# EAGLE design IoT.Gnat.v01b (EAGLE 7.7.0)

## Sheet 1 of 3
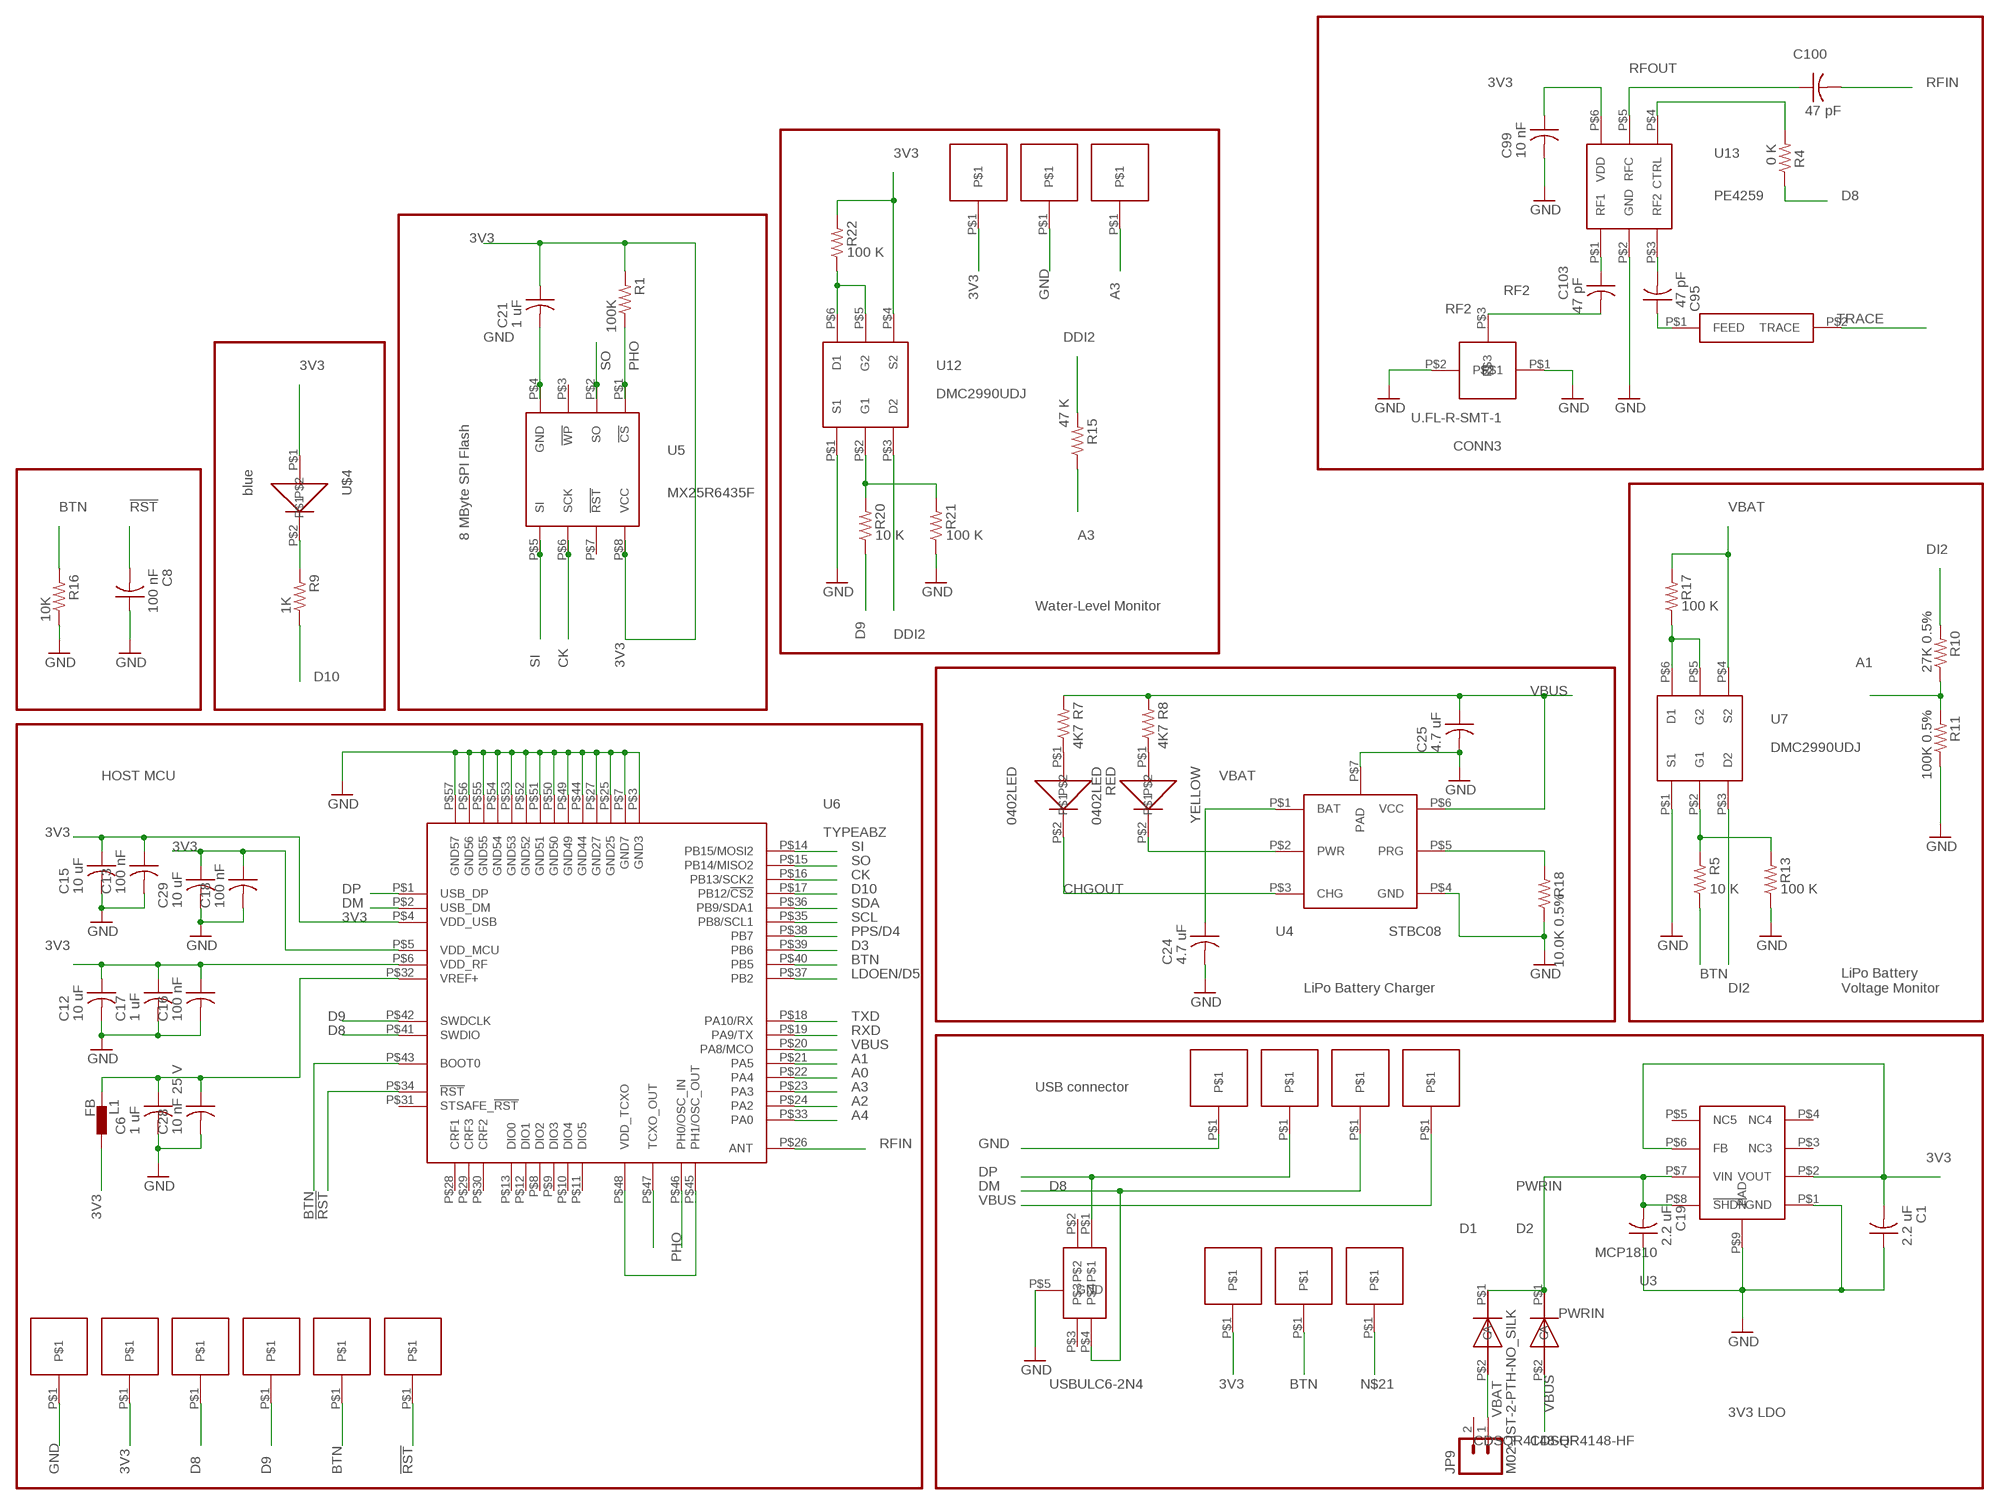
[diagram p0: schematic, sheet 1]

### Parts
C1  2.2 uF  C-US  [C0402_B]
C6  1 uF  C-US  [C0402_B]
C8  100 nF  C-US  [C0402_B]
C12  10 uF  C-US  [C0402_B]
C13  100 nF  C-US  [C0402_B]
C15  10 uF  C-US  [C0402_B]
C16  100 nF  C-US  [C0402_B]
C17  1 uF  C-US  [C0402_B]
C18  100 nF  C-US  [C0402_B]
C19  2.2 uF  C-US  [C0402_B]
C21  1 uF  C-US  [C0402_B]
C24  4.7 uF  C-US  [C0402_B]
C25  4.7 uF  C-US  [C0402_B]
C28  10 nF 25 V  C-US  [C0402_B]
C29  10 uF  C-US  [C0402_B]
C95  47 pF  C-US  [C0402_B]
C99  10 nF  C-US  [C0402_B]
C100  47 pF  C-US  [C0402_B]
C103  47 pF  C-US  [C0402_B]
CONN3  U.FL-R-SMT-1  [U.FL-R-SMT-1]
D1  CDSQR4148-HF  [CDSQR4148-HF]
D2  CDSQR4148-HF  [CDSQR4148-HF]
D8  USBULC6-2N4  [USBULC6-2N4]
JP9  M02-JST-2-PTH-NO_SILK  [JST-2-PTH-NS]
L1  FB  BLM15H  [0402]
R1  100K  R-US_  [R0402_B]
R4  0 K  R-US_  [R0402_B]
R5  10 K  R-US_  [R0402_B]
R7  4K7  R-US_  [R0402_B]
R8  4K7  R-US_  [R0402_B]
R9  1K  R-US_  [R0402_B]
R10  27K 0.5%  R-US_  [R0402_B]
R11  100K 0.5%  R-US_  [R0402_B]
R13  100 K  R-US_  [R0402_B]
R15  47 K  R-US_  [R0402_B]
R16  10K  R-US_  [R0402_B]
R17  100 K  R-US_  [R0402_B]
R18  10.0K 0.5%  R-US_  [R0402_B]
R20  10 K  R-US_  [R0402_B]
R21  100 K  R-US_  [R0402_B]
R22  100 K  R-US_  [R0402_B]
RED  0402LED  [0402LED]
U3  MCP1810  [MCP1810]
U4  STBC08  [STBC08]
U5  MX25R6435F  [MX25R6435F]
U6  TYPEABZ  [TYPEABZ]
U7  DMC2990UDJ  [DMC2990UDJ]
U12  DMC2990UDJ  [DMC2990UDJ]
U13  PE4259  [PE4259]
U$1  HN01  [HN01]
U$2  JOHANSON0900AT43A0070  [JOHANSON0900AT43A0070]
U$3  HN01  [HN01]
U$4  blue  0402LED  [0402LED]
U$6  HN01  [HN01]
U$7  HN01  [HN01]
U$8  HN01  [HN01]
U$9  HN01  [HN01]
U$10  HN01  [HN01]
U$11  HN01  [HN01]
U$12  HN01  [HN01]
U$13  HN01  [HN01]
U$14  HN01  [HN01]
U$15  HN01  [HN01]
U$16  HN01  [HN01]
U$17  HN01  [HN01]
U$18  HN01  [HN01]
U$19  HN01  [HN01]
YELLOW  0402LED  [0402LED]

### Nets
3V3: C1.2 C12.1 C13.1 C15.1 C16.1 C17.1 C18.1 C21.1 C29.1 C99.1 L1.2 R1.2 R22.2 U3.P$2(VOUT) U3.P$6(FB) U5.P$8(VCC) U6.P$4(VDD_USB) U6.P$5(VDD_MCU) U6.P$6(VDD_RF) U12.P$4(S2) U13.P$6(VDD) U$4.P$1 U$8.P$1 U$10.P$1 U$19.P$1 ; also sheet 2,3
!RST: C8.2 U6.P$34(!RST) U$9.P$1
A0: U6.P$22(PA4) ; also sheet 2
A1: R10.1 R11.2 U6.P$21(PA5)
A2: U6.P$24(PA2) ; also sheet 3
A3: R15.1 U6.P$23(PA3) U$12.P$1
A4: U6.P$33(PA0) ; also sheet 3
AREF: C6.1 C28.1 L1.1 U6.P$32(VREF+)
BTN: R5.1 R16.2 U6.P$40(PB5) U6.P$43(BOOT0) U$6.P$1 U$17.P$1
CHGOUT: RED.P$2 U4.P$3(CHG)
CK: U5.P$6(SCK) U6.P$16(PB13/SCK2)
D3: U6.P$39(PB6) ; also sheet 3
D8: R4.1 U6.P$41(SWDIO) U$1.P$1
D9: R20.1 U6.P$42(SWDCLK) U$3.P$1
D10: R9.1 U6.P$17(PB12/!CS2)
DDI2: R15.2 U12.P$3(D2)
DI2: R10.2 U7.P$3(D2)
DM: D8.P$4 U6.P$2(USB_DM) U$15.P$1
DP: D8.P$1 U6.P$1(USB_DP) U$14.P$1
GND: C1.1 C6.2 C8.1 C12.2 C13.2 C15.2 C16.2 C17.2 C18.2 C19.1 C21.2 C24.2 C25.2 C28.2 C29.2 C99.2 CONN3.P$1 CONN3.P$2 D8.P$5(GND) R11.1 R13.1 R16.1 R18.1 R21.1 U3.P$1(GND) U3.P$9(PAD) U4.P$4(GND) U4.P$7(PAD) U5.P$4(GND) U6.P$3(GND3) U6.P$7(GND7) U6.P$25(GND25) U6.P$27(GND27) U6.P$44(GND44) U6.P$49(GND49) U6.P$50(GND50) U6.P$51(GND51) U6.P$52(GND52) U6.P$53(GND53) U6.P$54(GND54) U6.P$55(GND55) U6.P$56(GND56) U6.P$57(GND57) U7.P$1(S1) U12.P$1(S1) U13.P$2(GND) U$7.P$1 U$11.P$1 U$13.P$1 ; also sheet 2,3
LDOEN/D5: U6.P$37(PB2) ; also sheet 2
N$2: U6.P$45(PH1/OSC_OUT) U6.P$48(VDD_TCXO)
N$3: R9.2 U$4.P$2
N$4: R20.2 R21.2 U12.P$2(G1)
N$7: U4.P$2(PWR) YELLOW.P$2
N$9: U6.P$47(TCXO_OUT)
N$10: R22.1 U12.P$5(G2) U12.P$6(D1)
N$12: R5.2 R13.2 U7.P$2(G1)
N$13: R17.1 U7.P$5(G2) U7.P$6(D1)
N$15: R7.1 RED.P$1
N$16: C95.1 U$2.P$1(FEED)
N$17: R8.1 YELLOW.P$1
N$18: C95.2 U13.P$3(RF2)
N$19: C103.1 U13.P$1(RF1)
N$21: U$18.P$1
N$22: R4.2 U13.P$4(CTRL)
N$27: R18.2 U4.P$5(PRG)
PHO: R1.1 U5.P$1(!CS) U6.P$46(PH0/OSC_IN)
PPS/D4: U6.P$38(PB7) ; also sheet 2
PWRIN: C19.2 D1.P$1(C) D2.P$1(C) U3.P$7(VIN) U3.P$8(!SHDN)
RF2: C103.2 CONN3.P$3
RFIN: C100.2 U6.P$26(ANT)
RFOUT: C100.1 U13.P$5(RFC)
RXD: U6.P$19(PA9/TX) ; also sheet 2
SCL: U6.P$35(PB8/SCL1) ; also sheet 3
SDA: U6.P$36(PB9/SDA1) ; also sheet 3
SI: U5.P$5(SI) U6.P$14(PB15/MOSI2)
SO: U5.P$2(SO) U6.P$15(PB14/MISO2)
TRACE: U$2.P$2(TRACE)
TXD: U6.P$18(PA10/RX) ; also sheet 2
VBAT: C24.1 D1.P$2(A) JP9.1 R17.2 U4.P$1(BAT) U7.P$4(S2)
VBUS: C25.1 D2.P$2(A) R7.2 R8.2 U4.P$6(VCC) U6.P$20(PA8/MCO) U$16.P$1
Unconnected: D8.P$2 D8.P$3 JP9.2 U3.P$3(NC3) U3.P$4(NC4) U3.P$5(NC5) U5.P$3(!WP) U5.P$7(!RST) U6.P$8(DIO2) U6.P$9(DIO3) U6.P$10(DIO4) U6.P$11(DIO5) U6.P$12(DIO1) U6.P$13(DIO0) U6.P$28(CRF1) U6.P$29(CRF3) U6.P$30(CRF2) U6.P$31(STSAFE_!RST)

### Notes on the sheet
- 8 MByte SPI Flash
- Water-Level Monitor
- HOST MCU
- LiPo Battery Charger
- LiPo Battery 
  Voltage Monitor
- USB connector
- 3V3 LDO

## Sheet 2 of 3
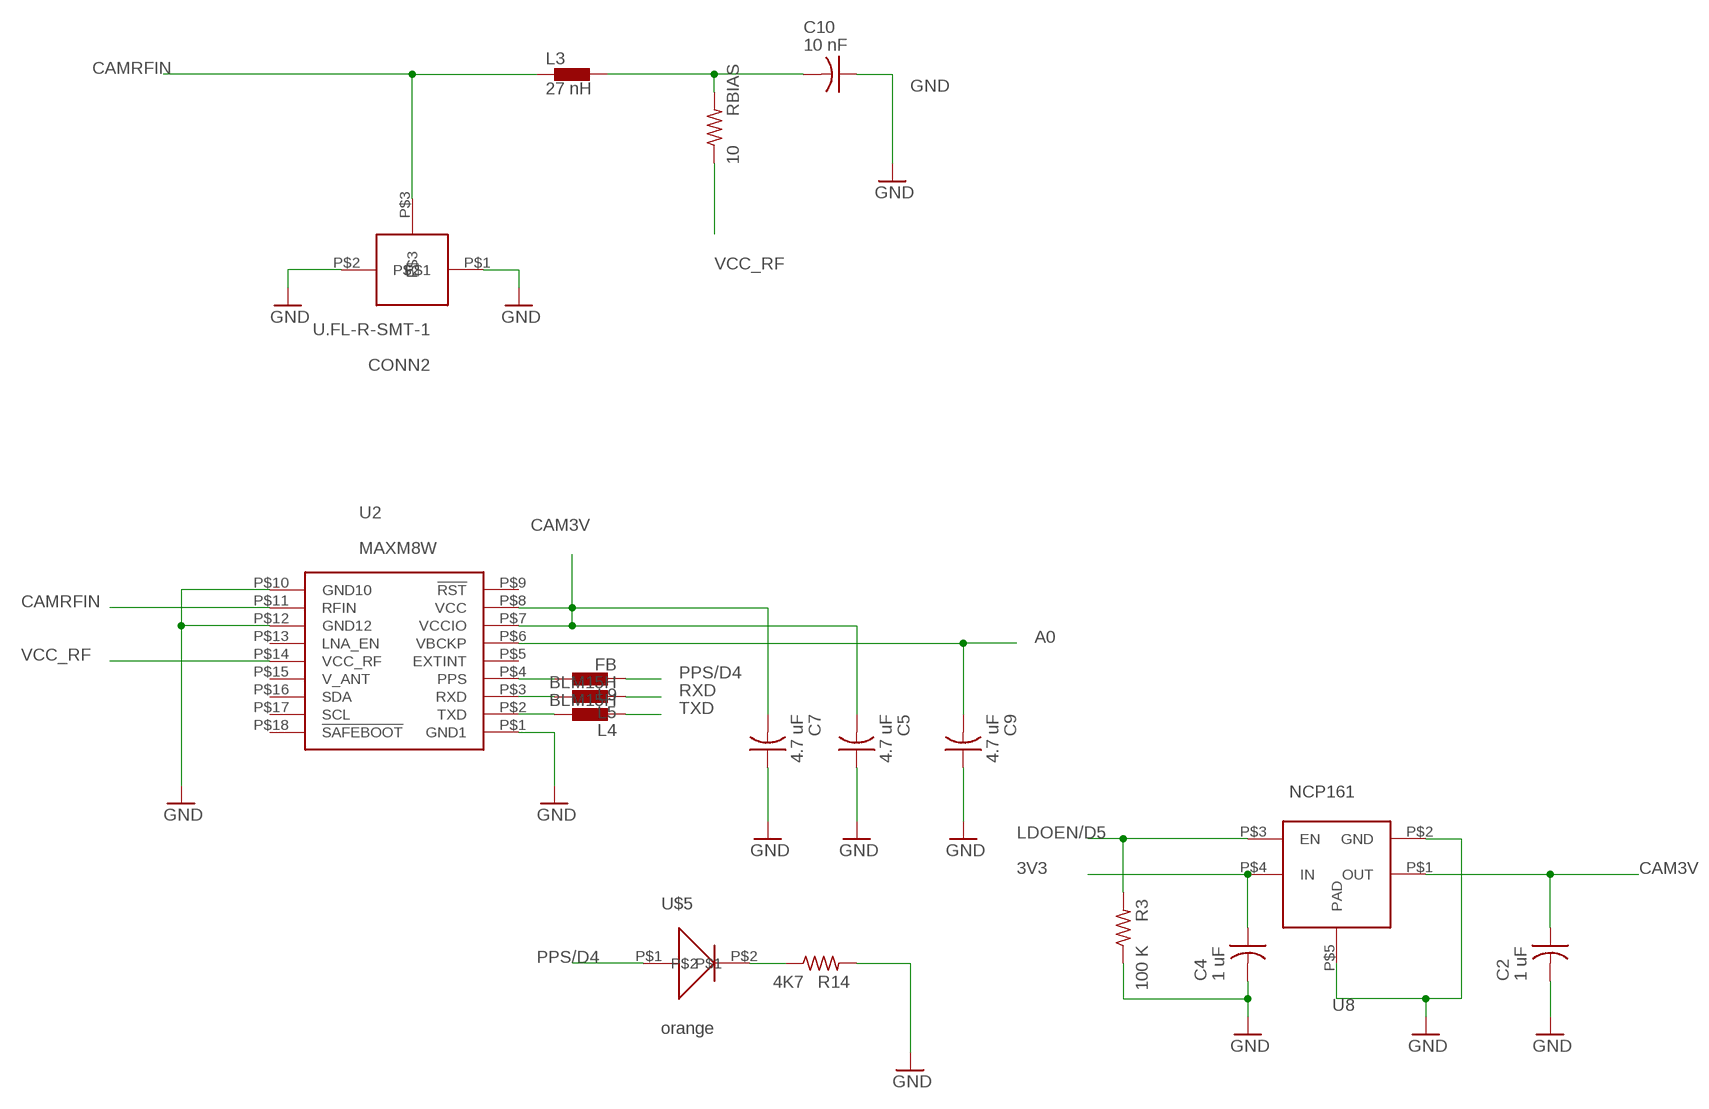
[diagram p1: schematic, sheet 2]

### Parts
C2  1 uF  C-US  [C0402_B]
C4  1 uF  C-US  [C0402_B]
C5  4.7 uF  C-US  [C0402_B]
C7  4.7 uF  C-US  [C0402_B]
C9  4.7 uF  C-US  [C0402_B]
C10  10 nF  C-US  [C0402_B]
CONN2  U.FL-R-SMT-1  [U.FL-R-SMT-1]
L3  27 nH  BLM15H  [0402]
L4  BLM15H  [0402]
L5  BLM15H  [0402]
L9  FB  BLM15H  [0402]
R3  100 K  R-US_  [R0402_B]
R14  4K7  R-US_  [R0402_B]
RBIAS  10  R-US_  [R0402_B]
U2  MAXM8W  [MAXM8W]
U8  NCP161  [NCP161]
U$5  orange  0402LED  [0402LED]

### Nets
3V3: C4.1 U8.P$4(IN) ; also sheet 1,3
A0: C9.2 U2.P$6(VBCKP) ; also sheet 1
CAM3V: C2.1 C5.2 C7.2 U2.P$7(VCCIO) U2.P$8(VCC) U8.P$1(OUT)
CAMRFIN: CONN2.P$3 L3.1 U2.P$11(RFIN)
GND: C2.2 C4.2 C5.1 C7.1 C9.1 C10.1 CONN2.P$1 CONN2.P$2 R3.1 R14.2 U2.P$1(GND1) U2.P$10(GND10) U2.P$12(GND12) U8.P$2(GND) U8.P$5(PAD) ; also sheet 1,3
LDOEN/D5: R3.2 U8.P$3(EN) ; also sheet 1
N$1: L9.2 U2.P$4(PPS)
N$5: C10.2 L3.2 RBIAS.2
N$8: R14.1 U$5.P$2
N$43: L4.2 U2.P$2(TXD)
N$44: L5.2 U2.P$3(RXD)
PPS/D4: L9.1 U$5.P$1 ; also sheet 1
RXD: L5.1 ; also sheet 1
TXD: L4.1 ; also sheet 1
VCC_RF: RBIAS.1 U2.P$14(VCC_RF)
Unconnected: U2.P$5(EXTINT) U2.P$9(!RST) U2.P$13(LNA_EN) U2.P$15(V_ANT) U2.P$16(SDA) U2.P$17(SCL) U2.P$18(!SAFEBOOT)

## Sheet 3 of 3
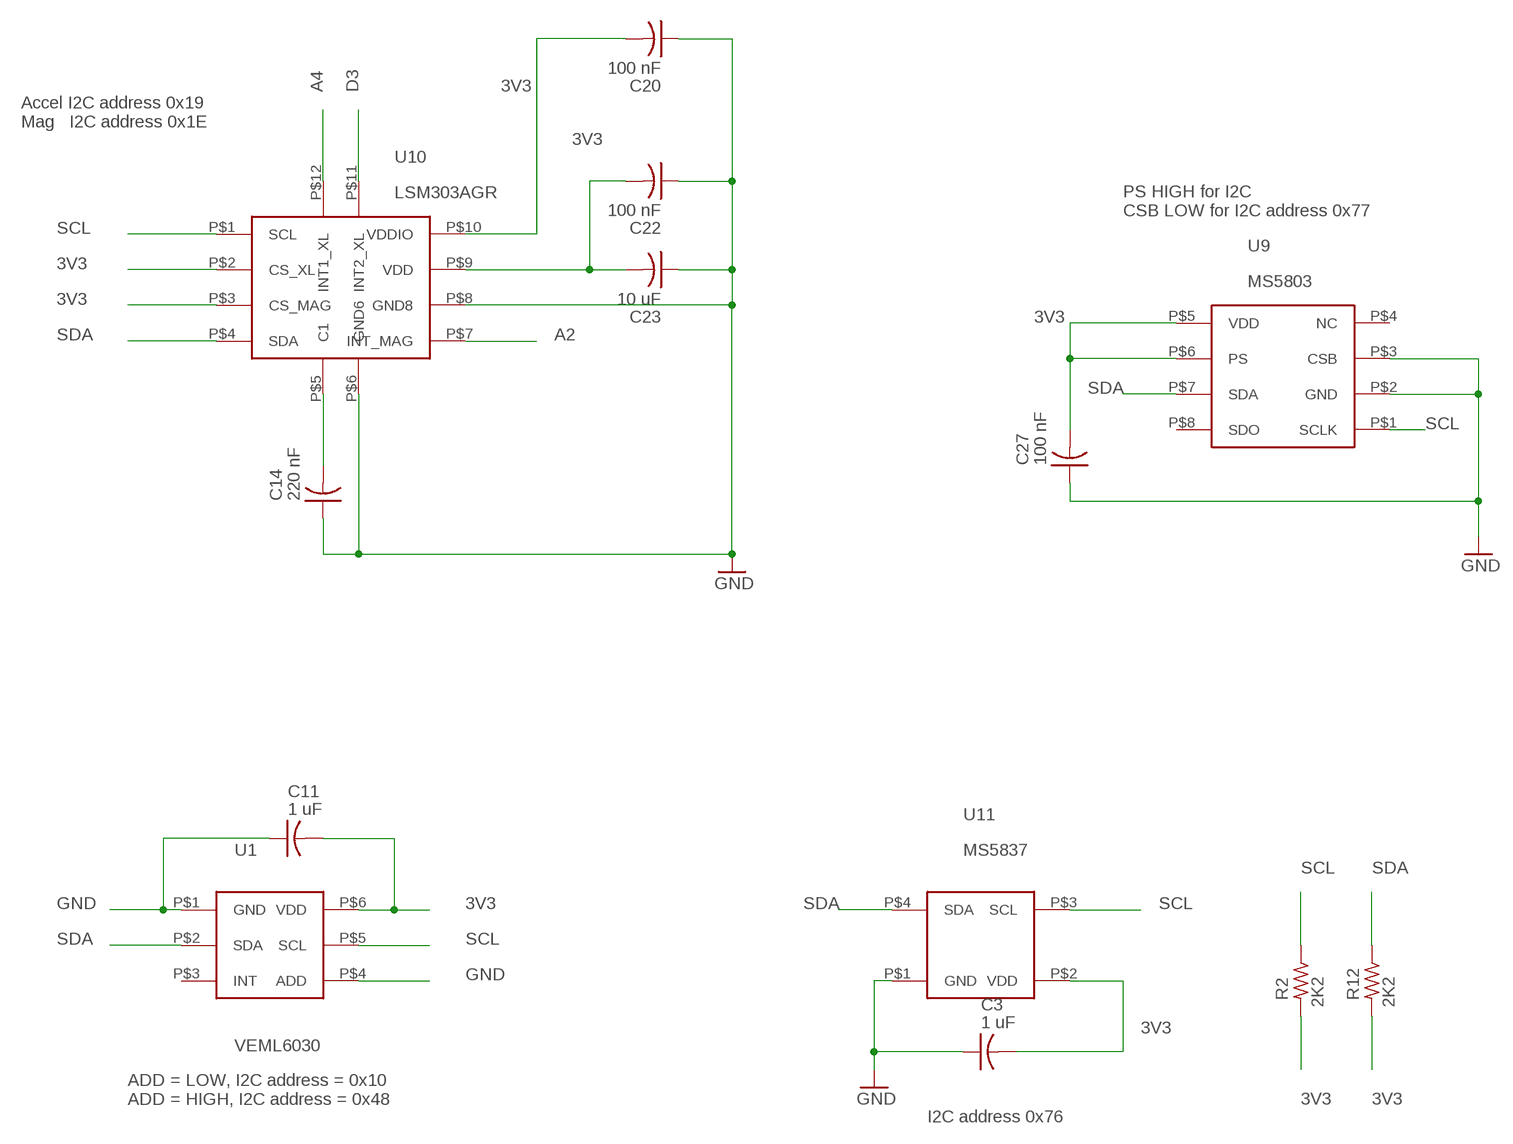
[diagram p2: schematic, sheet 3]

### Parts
C3  1 uF  C-US  [C0402_B]
C11  1 uF  C-US  [C0402_B]
C14  220 nF  C-US  [C0402_B]
C20  100 nF  C-US  [C0402_B]
C22  100 nF  C-US  [C0402_B]
C23  10 uF  C-US  [C0402_B]
C27  100 nF  C-US  [C0402_B]
R2  2K2  R-US_  [R0402_B]
R12  2K2  R-US_  [R0402_B]
U1  VEML6030  [VEML6030]
U9  MS5803  [MS5803]
U10  LSM303AGR  [LSM303AGR]
U11  MS5837  [MS5837]

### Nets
3V3: C3.2 C11.2 C20.2 C22.2 C23.2 C27.2 R2.2 R12.2 U1.P$6(VDD) U9.P$5(VDD) U9.P$6(PS) U10.P$2(CS_XL) U10.P$3(CS_MAG) U10.P$9(VDD) U10.P$10(VDDIO) U11.P$2(VDD) ; also sheet 1,2
A2: U10.P$7(INT_MAG) ; also sheet 1
A4: U10.P$12(INT1_XL) ; also sheet 1
D3: U10.P$11(INT2_XL) ; also sheet 1
GND: C3.1 C11.1 C14.1 C20.1 C22.1 C23.1 C27.1 U1.P$1(GND) U1.P$4(ADD) U9.P$2(GND) U9.P$3(CSB) U10.P$6(GND6) U10.P$8(GND8) U11.P$1(GND) ; also sheet 1,2
N$6: C14.2 U10.P$5(C1)
SCL: R2.1 U1.P$5(SCL) U9.P$1(SCLK) U10.P$1(SCL) U11.P$3(SCL) ; also sheet 1
SDA: R12.1 U1.P$2(SDA) U9.P$7(SDA) U10.P$4(SDA) U11.P$4(SDA) ; also sheet 1
Unconnected: U1.P$3(INT) U9.P$4(NC) U9.P$8(SDO)

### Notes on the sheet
- Accel I2C address 0x19
  Mag   I2C address 0x1E
- PS HIGH for I2C
  CSB LOW for I2C address 0x77
- ADD = LOW, I2C address = 0x10
  ADD = HIGH, I2C address = 0x48
- I2C address 0x76

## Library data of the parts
C1-C25 C27-C29 C95 C99 C100 C103 = Spark:C-US: Capacitor
CONN2 CONN3 = Kris:U.FL-R-SMT-1: U.FL-R-SMT-1
D1 D2 = Kris:CDSQR4148-HF: ComChip's CDSQR4148-HF high speed 150 mA Io diode
D8 = Kris:USBULC6-2N4: ST TVS diode ESD Protection USBULC6-2N4
JP9 = SparkFun-Connectors:M02: Standard 2-pin 0.1" header. Use with
L1 L3-L5 L9 = STM32L433SARA.AssetTracker.v01:BLM15H: EMIFIL (R) Chip Ferrite Bead for GHz Noise
R1-R5 R7-R18 R20-R22 RBIAS = Spark:R-US_: 0402 Resistor
RED U$4 U$5 YELLOW = Kris:0402LED: 0402led
U1 = Kris:VEML6030: VEML6030 ambient light sensor https://www.vishay.com/docs/84366/veml6030.pdf
U2 = Kris:MAXM8W: MAX M8W Concurrent GNSS Module https://www.u-blox.com/sites/default/files/MAX-8-M8-FW3_HardwareIntegrationManual_%28UBX-15030059%29.pdf
U3 = Kris:MCP1810: MCP1810 3.0 V Low Iq LDO http://ww1.microchip.com/downloads/en/DeviceDoc/20005623A.pdf
U4 = Kris:STBC08: STBC08
U5 = Kris:MX25R6435F: MX25R6435F 64 MBit SPI NOR Flash from Macronix
U6 = Kris:TYPEABZ: CMWX1ZZABZ-078
U7 U12 = Kris:DMC2990UDJ: DMC2990UDJ dual N-Type and P-Type MOSFET COMPLEMENTARY PAIR ENHANCEMENT MODE MOSFET https://www.diodes.com/assets/Datasheets/DMC2990UDJ.pdf
U8 = Kris:NCP161: NCP161 3V3 LDO voltage regulator
U9 = Kris:MS5803: MS5803 barometer https://cdn.sparkfun.com/datasheets/Sensors/Weather/ms5803_14ba.pdf
U10 = Kris:LSM303AGR: LSM303AGR e-compass
U11 = Kris:MS5837: MS5837 pressure sensor
U13 = Kris:PE4259: PE4259 RF switch http://www.psemi.com/pdf/datasheets/pe4259ds.pdf
U$1 U$3 U$6-U$19 = PWSONN6:HN01
U$2 = Kris:JOHANSON0900AT43A0070: Johanson dual wide band antenna

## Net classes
1 USB: width 0.254 mm, drill 0.33 mm, clearance 0.159 mm
2 Top GND Pour: clearance 0.762 mm to class 1

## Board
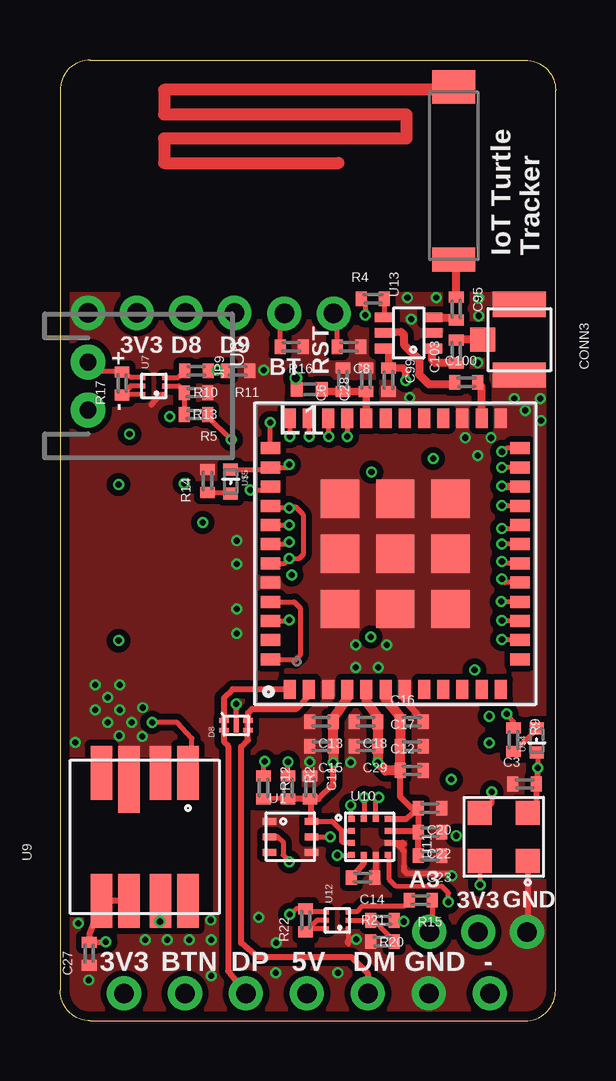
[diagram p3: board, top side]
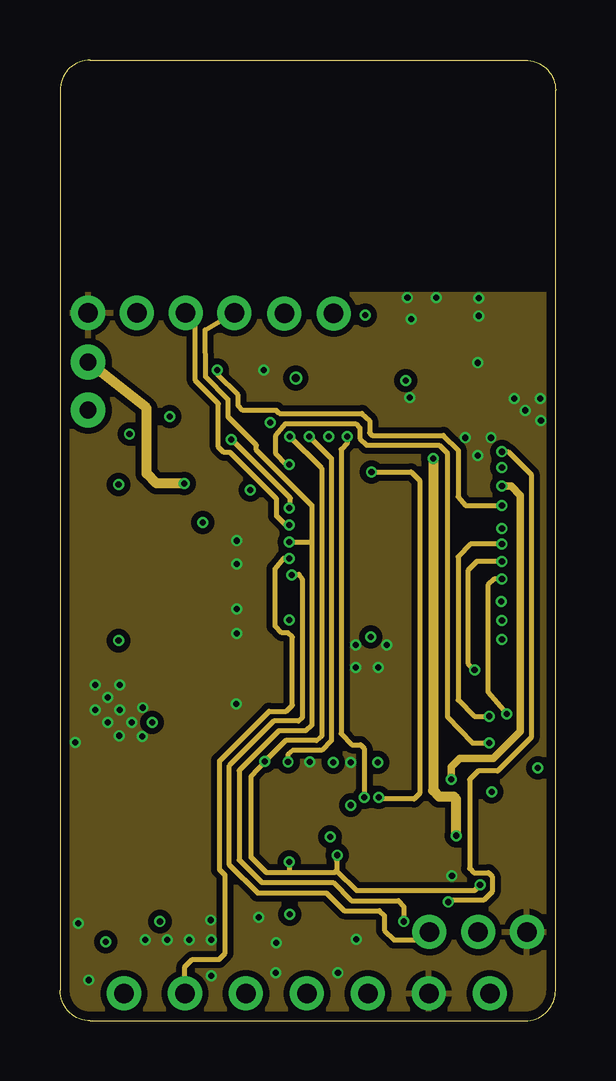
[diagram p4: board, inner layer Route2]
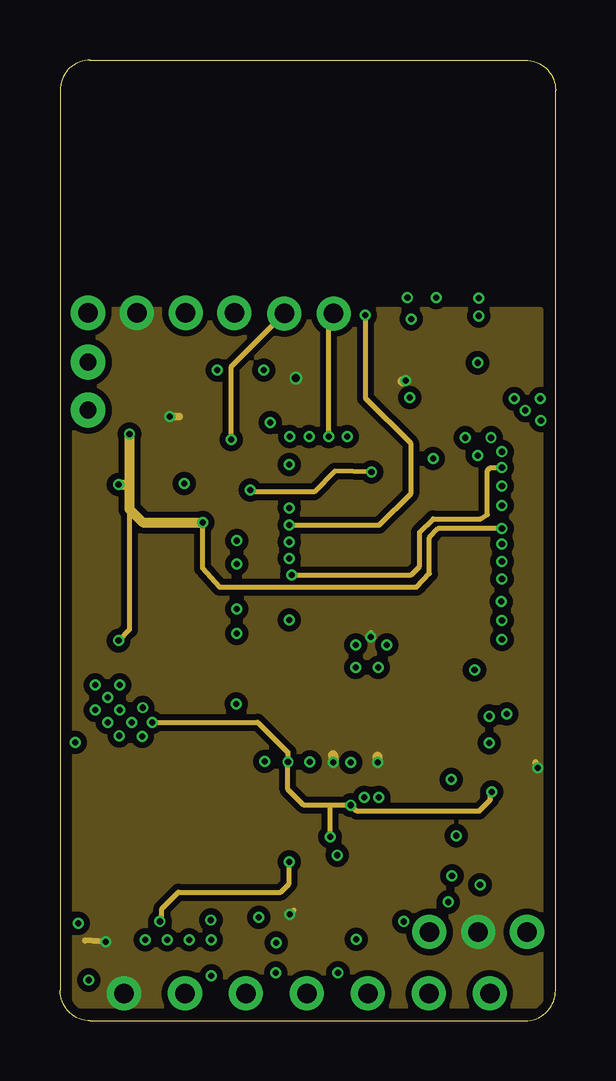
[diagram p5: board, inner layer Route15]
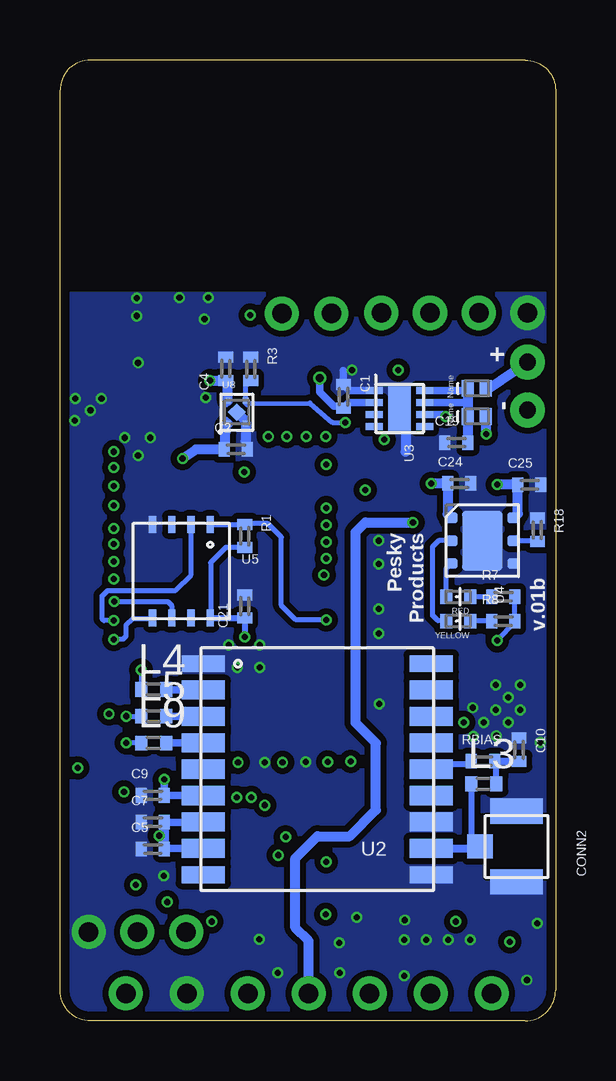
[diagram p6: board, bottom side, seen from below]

Size 20.65 x 40.06 mm. Coordinates in mm from the lower left corner, seen from the top.
Outline: 1.27,0 19.38,0 arc90 20.65,1.27 20.65,38.79 arc90 19.38,40.06 1.27,40.06 arc90 0,38.79 0,1.27 arc90 1.27,0
Copper layers (1*2*15*16): Top 0.035559375mm / dielectric 0.17018125mm / Route2 0.01778125mm / dielectric 47mil / Route15 0.01778125mm / dielectric 0.17018125mm / Bottom 0.035559375mm
Design rules "OSHPark-4layer *": minimum track width 5mil, minimum drill 10mil, track to track 5mil, track to pad 5mil, pad to pad 5mil, via to via 5mil, smd to smd 5mil, copper to edge 15mil, drill to drill 6mil, minimum pad ring 4mil, minimum via ring 4mil, stop-mask expansion 4mil, vias tented up to drill 20mil, thermal gap 10mil

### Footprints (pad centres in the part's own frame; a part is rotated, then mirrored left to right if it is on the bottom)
C0402_B = smd 0.457 x 0.61: 1 -0.483,0; 2 0.483,0
U.FL-R-SMT-1 = smd 1.05 x 2.2: P$1 -1.475,0; P$2 1.475,0 | smd 1 x 1.05: P$3 0,-1.525
CDSQR4148-HF = smd 0.7 x 0.5: P$1 0,0.375; P$2 0,-0.375
USBULC6-2N4 = smd 0.2 x 0.4: P$1 0.2,0.5; P$2 -0.2,0.5; P$3 -0.2,-0.5; P$4 0.2,-0.5 | smd 0.6 x 0.2: P$5 0,0
JST-2-PTH-NS = drill 0.7 pad 1.448: 1 -1,0; 2 1,0
0402 = smd 0.5 x 0.61: 1 -0.5,0; 2 0.55,0
R0402_B = smd 0.457 x 0.61: 1 -0.483,0; 2 0.483,0
0402LED = smd 0.5 x 0.6: P$1 -0.5,0; P$2 0.5,0
VEML6030 = smd 0.55 x 0.3: P$1 -0.875,0.65; P$2 -0.875,0; P$3 -0.875,-0.65; P$4 0.875,-0.65; P$5 0.875,0; P$6 0.875,0.65
MAXM8W = smd 1.8 x 0.7: P$1 4.75,-4.4; P$9 4.75,4.4; P$10 -4.75,4.4; P$18 -4.75,-4.4 | smd 1.8 x 0.8: P$2 4.75,-3.3; P$3 4.75,-2.2; P$4 4.75,-1.1; P$5 4.75,0; P$6 4.75,1.1; P$7 4.75,2.2; P$8 4.75,3.3; P$11 -4.75,3.3; P$12 -4.75,2.2; P$13 -4.75,1.1; P$14 -4.75,0; P$15 -4.75,-1.1; P$16 -4.75,-2.2; P$17 -4.75,-3.3
MCP1810 = smd 0.3 x 0.7: P$1 -0.75,-1.05; P$2 -0.25,-1.05; P$3 0.25,-1.05; P$4 0.75,-1.05; P$5 0.75,1.05; P$6 0.25,1.05; P$7 -0.25,1.05; P$8 -0.75,1.05 | smd 1.95 x 0.95: P$9 0,0
STBC08 = smd 0.45 x 0.5: P$1 -0.95,-1.3; P$2 0,-1.3; P$3 0.95,-1.3; P$4 0.95,1.3; P$5 0,1.3; P$6 -0.95,1.3 | smd 2.5 x 1.69: P$7 0,0
MX25R6435F = smd 0.3 x 0.7: P$1 1.2,1.95; P$2 0.4,1.95; P$3 -0.4,1.95; P$4 -1.2,1.95; P$5 -1.2,-1.95; P$6 -0.4,-1.95; P$7 0.4,-1.95; P$8 1.2,-1.95
TYPEABZ = smd 0.8 x 0.5: P$1 -5.65,4.4; P$2 -5.65,3.6; P$3 -5.65,2.8; P$4 -5.65,2; P$5 -5.65,1.2; P$6 -5.65,0.4; P$7 -5.65,-0.4; P$8 -5.65,-1.2; P$9 -5.65,-2; P$10 -5.65,-2.8; P$11 -5.65,-3.6; P$12 -5.65,-4.4; P$25 5.65,-4.4; P$26 5.65,-3.6; P$27 5.65,-2.8; P$28 5.65,-2; P$29 5.65,-1.2; P$30 5.65,-0.4; P$31 5.65,0.4; P$32 5.65,1.2; P$33 5.65,2; P$34 5.65,2.8; P$35 5.65,3.6; P$36 5.65,4.4 | smd 0.5 x 0.8: P$13 -4.4,-5.2; P$14 -3.6,-5.2; P$15 -2.8,-5.2; P$16 -2,-5.2; P$17 -1.2,-5.2; P$18 -0.4,-5.2; P$19 0.4,-5.2; P$20 1.2,-5.2; P$21 2,-5.2; P$22 2.8,-5.2; P$23 3.6,-5.2; P$24 4.4,-5.2; P$37 4.4,5.2; P$38 3.6,5.2; P$39 2.8,5.2; P$40 2,5.2; P$41 1.2,5.2; P$42 0.4,5.2; P$43 -0.4,5.2; P$44 -1.2,5.2; P$45 -2,5.2; P$46 -2.8,5.2; P$47 -3.6,5.2; P$48 -4.4,5.2 | smd 1.6 x 1.6: P$49 -2.3,2.3; P$50 0,2.3; P$51 2.3,2.3; P$52 -2.3,0; P$53 0,0; P$54 2.3,0; P$55 -2.3,-2.3; P$56 0,-2.3; P$57 2.3,-2.3
DMC2990UDJ = smd 0.2 x 0.2: P$1 -0.35,-0.45; P$2 0,-0.45; P$3 0.35,-0.45; P$4 0.35,0.45; P$5 0,0.45; P$6 -0.35,0.45
NCP161 = smd 0.24 x 0.24: P$1 -0.37,-0.48; P$2 0.37,-0.48; P$3 0.37,0.48; P$4 -0.37,0.48 | smd 0.52 x 0.52 rotated 45: P$5 0,0
MS5803 = smd 2.25 x 0.9: P$1 2.675,-1.8; P$2 2.675,-0.65; P$4 2.675,1.8; P$5 -2.675,1.8; P$6 -2.675,0.65; P$7 -2.675,-0.65; P$8 -2.675,-1.8 | smd 2.8 x 0.9: P$3 2.4,0.65
LSM303AGR = smd 0.275 x 0.25: P$1 -0.762,0.75; P$2 -0.762,0.25; P$3 -0.762,-0.25; P$4 -0.762,-0.75; P$7 0.762,-0.75; P$8 0.762,-0.25; P$9 0.762,0.25; P$10 0.762,0.75 | smd 0.25 x 0.275: P$5 -0.25,-0.762; P$6 0.25,-0.762; P$11 0.25,0.762; P$12 -0.25,0.762
MS5837 = smd 1 x 1: P$1 -1,-1; P$2 1,-1; P$3 1,1; P$4 -1,1
PE4259 = smd 0.4 x 0.8: P$1 -0.65,-1; P$2 0,-1; P$3 0.65,-1; P$4 0.65,1; P$5 0,1; P$6 -0.65,1
HN01 = drill 0.813 pad 1.422: P$1 0,0
JOHANSON0900AT43A0070 = smd 1 x 1.8: P$1 -3.5,0 | smd 1.4 x 1.8: P$2 3.7,0

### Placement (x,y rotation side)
C1  8.84,26.04 270 bottom
C2  13.32,23.82 0 bottom
C3  19.35,9.88 0 top
C4  13.74,27.18 90 bottom
C5  16.79,7.16 0 bottom
C6  11.79,26.72 90 top
C7  16.79,8.28 0 bottom
C8  12.04,28.09 180 top
C9  16.79,9.4 0 bottom
C10  1.52,11.3 270 bottom
C11  10.41,9.73 270 top
C12  14.66,10.44 0 top
C13  10.9,12.47 180 top
C14  12.62,5.97 180 top
C15  10.9,11.46 180 top
C16  14.66,12.47 0 top
C17  14.66,11.46 0 top
C18  12.75,12.47 180 top
C19  4.14,24.1 0 bottom
C20  15.42,8.86 180 top
C21  12.95,17.27 90 bottom
C22  15.42,7.87 180 top
C23  15.42,6.88 180 top
C24  4.01,22.4 0 bottom
C25  1.09,22.35 0 bottom
C27  1.22,2.79 90 top
C28  12.75,26.72 90 top
C29  12.75,11.46 180 top
C95  16.51,29.69 270 top
C99  13.69,26.72 270 top
C100  16.93,26.62 0 top
C103  16.51,27.9 90 top
CONN2  1.63,7.26 270 bottom
CONN3  19.14,28.4 270 top
D1  3.28,26.37 90 bottom
D2  3.28,25.2 90 bottom
D8  7.34,12.32 90 top
JP9  1.17,26.47 270 top
L1  10.41,26.33 180 top
L3  3.02,9.88 0 bottom
L4  16.76,13.82 0 bottom
L5  16.76,12.7 0 bottom
L9  16.76,11.58 0 bottom
R1  12.95,20.22 270 bottom
R2  9.5,9.73 270 top
R3  12.7,27.18 270 bottom
R4  13.03,30.1 0 top
R5  5.66,25.27 180 top
R7  2.18,17.68 0 bottom
R8  2.18,16.66 0 bottom
R9  18.9,11.72 270 top
R10  5.69,27.1 180 top
R11  7.42,27.1 180 top
R12  8.48,9.73 270 top
R13  5.66,26.19 180 top
R14  6.15,22.5 90 top
R15  15.04,5.03 180 top
R16  9.65,28.09 180 top
R17  2.59,26.57 90 top
R18  0.76,20.47 270 bottom
R20  13.44,4.19 180 top
R21  13.44,3.3 0 top
R22  10.24,4.19 90 top
RBIAS  3.02,10.82 0 bottom
RED  4.06,17.68 180 bottom
U1  9.6,7.67 0 top
U2  9.93,10.49 180 bottom
U3  6.5,25.53 270 bottom
U4  3.05,20.02 270 bottom
U5  15.6,18.75 0 bottom
U6  13.97,19.47 90 top
U7  3.91,26.47 90 top
U8  13.28,25.37 0 bottom
U9  3.53,7.67 90 top
U10  12.9,7.67 0 top
U11  18.49,7.67 90 top
U12  11.56,4.19 90 top
U13  14.52,28.68 90 top
U$1  5.23,29.51 0 top
U$2  16.41,35.23 90 top
U$3  7.26,29.51 0 top
U$4  19.86,11.68 90 top
U$5  7.11,22.48 270 top
U$6  9.35,29.49 0 top
U$7  1.17,29.51 0 top
U$8  3.2,29.51 0 top
U$9  11.4,29.49 0 top
U$10  17.42,3.71 0 top
U$11  19.46,3.71 0 top
U$12  15.39,3.71 0 top
U$13  15.37,1.14 0 top
U$14  7.75,1.14 0 top
U$15  12.83,1.14 0 top
U$16  10.29,1.14 0 top
U$17  5.21,1.14 0 top
U$18  17.91,1.14 0 top
U$19  2.67,1.14 0 top
YELLOW  4.06,16.66 180 bottom

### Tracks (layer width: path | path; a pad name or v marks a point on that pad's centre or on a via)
3V3  (via drill 0.25, 0.33)
  Top 0.203: U$4.P$1 19.91,11.09 v19.91,10.54 | R2.2 8.51,9.27 | U1.P$6 11.34,8.32 11.63,8.03 | 11.63,8.03 11.78,7.92 U10.P$2 | U10.P$3 11.83,7.42 11.73,7.47 11.73,7.92 11.63,8.03 | U12.P$4 10.39,4.54 R22.2 9.86,4.67 v9.58,4.44
  Top 0.254: v19.91,10.54 19.91,10.01 C3.2 19.84,8.86 | U10.P$9 14.91,7.92 C22.2 | C23.2 C22.2 | C20.2 14.66,8.86 14.17,9.35 C12.1 | C20.2 C22.2 | U10.P$10 14.44,8.42 C20.2 | v11.38,10.77 11.38,9.85 10.77,9.25 C11.2 | U1.P$6 10.48,9.16 C11.2 | C11.2 R2.2 | 8.51,9.27 R12.2 | U9.P$6 U9.P$5 1.22,3.61 C27.2 v1.91,3.3
  Top 0.305: 14.17,12.55 C16.1 | 14.17,11.53 C17.1 | 11.38,12.45 C13.1 | L1.2 9.86,26.5 v9.83,26.8 | 19.84,8.86 U11.P$2 | U13.P$6 13.69,27.91 C99.1 14.3,27.2 14.4,27.08 v14.4,26.7
  Top 0.406: U6.P$4 11.97,13.47 11.38,12.6 C13.1 | U6.P$6 13.57,13.4 14.17,12.65 14.17,12.55 C17.1 C12.1 13.56,10.44 v13.23,10.77 C29.1 C18.1 13.23,12.65 12.77,13.34 U6.P$5 | 11.38,12.45 C15.1 v11.38,10.77
  Route15 0.203: v9.58,4.44 9.75,4.62
  Route15 0.254: v19.91,10.54 19.81,10.79 | v12.95,16 12.95,16.15 | v1.91,3.3 1.04,3.35
  Route15 0.305: v9.83,26.8 9.86,26.75 | v4.57,25.2 4.98,25.2
  Route15 0.406: v13.23,10.77 13.23,11.02 | 11.38,11.07 v11.38,10.77 | v14.4,26.7 14.28,26.67
  Bottom 0.203: R1.2 13.74,19.74 14.38,19.1 14.38,16.81 U5.P$8
  Bottom 0.254: U5.P$8 C21.1 v12.95,16
  Bottom 0.305: U3.P$6 4.72,25.28 v4.57,25.2 | U3.P$2 8.62,25.78 C1.2 8.89,25.55 9.07,25.63 9.25,25.63 9.83,26.21 v9.83,26.8
  Bottom 0.406: U8.P$4 13.65,26.58 C4.1 v14.4,26.7
  pour Route15 (isolate 0.254, no thermals): 0.64,0.63 0.64,29.64 20.02,29.64 20.02,0.63
!RST  (via drill 0.25)
  Top 0.203: U6.P$34 11.17,24.34 v11.2,24.36 | C8.2 11.56,29.34 U$9.P$1
  Route15 0.203: v11.2,24.36 11.2,29.29 U$9.P$1
A0  (via drill 0.25)
  Top 0.203: 18.55,22.27 v18.41,22.3
  Top 0.305: U6.P$22 18.55,22.27
  Route2 0.305: v18.41,22.3 18.8,22.3 19.18,21.89 19.18,12.06 18.06,10.95 16.66,10.95 16.31,10.59 v16.31,10.06
  Bottom 0.305: U2.P$6 C9.2 v16.31,10.06
A1  (via drill 0.25)
  Top 0.203: U6.P$21 18.53,21.47 v18.41,21.49 | R10.1 6.3,26.97 v6.55,27.13 6.83,26.97 R11.2
  Route2 0.203: v18.41,21.49 16.89,21.49 16.59,21.84 16.59,23.8 15.98,24.41 13,24.41 12.9,24.51 12.9,25.02 12.57,25.32 9.14,25.32 9.02,25.45 7.62,25.45 7.42,25.65 7.42,26.09 6.55,26.95 v6.55,27.13
A2  (via drill 0.25)
  Top 0.203: U6.P$24 18.62,23.87 v18.41,23.72 | U10.P$7 13.7,6.88 13.7,5.91 13.97,5.64 15.9,5.61 16.18,5.33 v16.18,4.95
  Route2 0.203: v18.41,23.72 18.67,23.72 19.63,22.78 19.63,11.81 18.24,10.41 17.42,10.41 17.07,10.06 17.07,6.35 17.25,6.17 17.86,6.17 18.01,6.02 18.01,5.38 17.65,5.03 16.28,5.03 v16.18,4.95
A3  (via drill 0.25)
  Top 0.203: 19.16,23.06 U6.P$23 18.46,23.07 v18.41,23.06 | R15.1 15.52,3.84 U$12.P$1
  Route2 0.203: 9.73,18.62 9.96,18.62 10.08,18.41 10.08,12.62 9.93,12.5 8.91,12.5 7.06,10.64 7.06,6.5 8.23,5.33 11.1,5.33 11.84,4.6 13.31,4.6 13.51,4.39 13.51,3.78 13.92,3.38 15.06,3.38 U$12.P$1
  Route2 0.254: 9.73,18.62 v9.65,18.59
  Route15 0.203: v9.65,18.59 14.63,18.59 14.99,18.95 14.99,20.37 15.55,20.93 17.53,20.93 17.8,21.11 17.8,22.94 17.93,23.06 v18.41,23.06
A4  (via drill 0.25)
  Top 0.203: U6.P$33 11.97,24.54 v11.96,24.36 | v12.68,9.32 12.68,8.48 U10.P$12
  Route2 0.203: v11.96,24.36 11.96,24.08 11.71,23.82 11.71,11.96 12.17,11.51 12.52,11.51 12.68,11.35 v12.68,9.32
AREF
  Top 0.254: L1.1 10.85,26.24 | C28.1 12.75,26.22 12.77,26.2
  Top 0.305: U6.P$32 12.77,26.2 | C28.1 C6.1 10.85,26.24
BTN  (via drill 0.25)
  Top 0.203: R5.1 6.15,25.2 v7.14,24.23 | 8.76,21.46 U6.P$40 8.86,21.39 v9.55,21.39 9.5,21.41 9.83,21.41 10.14,21.11 10.14,19.43 9.98,19.27 9.73,19.27 v9.55,19.28 9.35,19.07 U6.P$43 | R16.2 9.17,29.31 U$6.P$1
  Route2 0.203: v7.14,24.23 7.14,24.26 9.6,21.79 9.6,21.39 v9.55,21.39 | U$17.P$1 5.21,2.26 5.51,2.57 6.63,2.57 6.88,2.82 6.88,6.07 6.66,6.3 6.66,10.85 8.71,12.9 9.42,12.9 9.68,13.16 9.68,16 9.5,16.18 9.25,16.18 8.97,16.46 8.97,18.85 9.32,19.28 v9.55,19.28
  Route15 0.203: v7.14,24.23 7.14,27.28 U$6.P$1
CAM3V  (via drill 0.25)
  Route2 0.406: v15.55,23.44 15.55,9.6 15.8,9.35 16.41,9.35 16.51,9.25 v16.51,7.72
  Bottom 0.305: U2.P$8 16.3,7.19 C5.2 | C7.2 14.69,8.28 U2.P$7
  Bottom 0.406: U8.P$1 13.76,24.8 13.77,24.69 C2.1 14.98,23.82 v15.55,23.44 | 16.31,7.7 C7.2 | C5.2 16.31,7.7 | 16.31,7.7 v16.51,7.72
CAMRFIN
  Bottom 0.254: L3.1 3.52,7.51 CONN2.P$3
  Bottom 0.305: 3.38,7.19 CONN2.P$3
  Bottom 0.33: U2.P$11 3.38,7.19
CHGOUT
  Bottom 0.203: RED.P$2 4.56,18.85 U4.P$3
CK  (via drill 0.25)
  Top 0.203: U6.P$16 18.5,17.47 v18.39,17.47
  Bottom 0.203: v18.39,17.47 16.15,17.47 16,17.32 U5.P$6
D3  (via drill 0.25)
  Top 0.203: v7.93,22.12 8.51,22.12 U6.P$39 | U10.P$11 13.15,9.24 v13.28,9.32
  Route2 0.203: v12.98,22.89 14.63,22.89 14.99,22.53 14.99,9.47 14.76,9.25 13.36,9.25 v13.28,9.32
  Route15 0.203: v12.98,22.89 11.46,22.91 10.59,22.05 7.98,22.05 v7.93,22.12
D8  (via drill 0.25)
  Top 0.203: U6.P$41 8.56,20.67 v9.55,20.68 | R4.1 12.74,29.96 12.74,29.48 v12.73,29.41
  Route2 0.203: U$1.P$1 5.64,29.06 5.64,26.7 6.6,25.73 6.6,23.93 6.83,23.7 7.09,23.7 9.02,21.77 9.02,21.06 9.4,20.68 v9.55,20.68
  Route15 0.203: v12.73,29.41 12.73,25.96 14.61,24.08 14.61,21.97 13.28,20.65 9.58,20.65 v9.55,20.68
D9  (via drill 0.25)
  Top 0.203: U6.P$42 9.52,19.87 v9.55,19.96 | v14.33,4.14 14.25,4.11 R20.1
  Route2 0.203: v14.33,4.14 14.33,4.75 14.1,5 12.14,5 11.38,5.77 8.41,5.77 7.47,6.71 7.47,10.44 9.12,12.09 10.24,12.09 10.49,12.32 10.49,19.96 | 10.49,19.96 10.49,21.49 8.18,23.8 8.18,24 7.01,25.17 7.01,25.91 6.07,26.85 6.05,28.8 U$3.P$1 | v9.55,19.96 10.49,19.96
D10  (via drill 0.25)
  Top 0.203: U6.P$17 18.53,18.27 v18.41,18.41 | 18.9,12.19 R9.1 18.9,12.47 v18.61,12.8
  Route2 0.203: v18.41,18.41 18.09,18.41 17.83,18.16 17.83,13.72 v18.61,12.8
DDI2
  Top 0.203: 12.03,4.52 U12.P$3 12.37,4.55 12.57,4.77 14.35,4.77 14.55,4.93 R15.2
DI2
  Top 0.203: U7.P$3 4.92,26.82 R10.2
DM
  Top 0.203: U6.P$2 10.37,13.52
  Top 0.254: 10.37,13.52 9.86,13 8,13 7.84,12.84 D8.P$4 7.82,12.5 7.82,11.71 7.54,11.43 7.54,3.25 8.23,2.67 12.14,2.67 12.83,1.98 U$15.P$1
DP
  Top 0.254: U6.P$1 7.19,13.82 6.83,13.46 6.83,12.53 | U$14.P$1 7.06,2.03 7.01,2.08 7.01,11.46 6.83,11.63 6.83,12.53 | 6.83,12.53 D8.P$1
GND  (via drill 0.25)
  Top 0.203: U7.P$1 4.18,26.09 | U12.P$1 12.01,3.29 12.01,3.2 | 14.33,7.09 14.33,6.45 | D8.P$5 v7.34,13.21
  Top 0.254: 4.18,26.09 3.81,25.68 | 14.33,7.09 14.07,7.37 U10.P$8 14.27,7.42 14.33,7.37 | C14.1 13.15,5.96 U10.P$6 13.15,6.02 13.13,5.99 | U11.P$1 19.49,3.74 U$11.P$1 | v12.34,3.4 12.12,3.4 11.99,3.28 | 14.33,6.45 14.33,6.27 14.45,6.15 16.18,6.15 v16.33,6.04
  Top 0.305: U6.P$7 14.37,13.39 C16.2
  Bottom 0.305: U3.P$1 8.6,26.28 C1.1 8.84,27.1
  Bottom 0.406: U8.P$5 12.95,25.04 U8.P$2 12.91,24.17 C2.2 | U3.P$9 6.5,25.3 6.25,25.04 6.25,23.72
  other vias: 12.12,10.77 19.38,25.45 13.26,14.73 12.32,14.73 8.48,27.13 16.89,24.31 10.41,10.79 13.61,15.67 12.32,15.67 7.37,20.02 7.37,19.05 7.37,17.17 7.37,16.15 18.92,25.93 20.02,25.93 20.04,25.02 14.58,25.98 0.64,11.61 2.46,11.89 3.43,11.86 8.99,2.01 6.29,4.2 3.56,3.38 4.47,3.38 5.38,3.38 8.28,4.32 9.02,3.25 6.3,3.38 6.3,1.88 3.45,13.06 1.98,13.49 1.47,14 2.49,14 1.98,12.45 3,12.45 1.47,12.95 2.49,12.95 0.76,4.06 15.67,30.15 14.48,30.15 14.63,29.26 17.45,30.12 17.4,27.43 11.58,2.01 17.45,29.39 1.19,1.7 17.96,24.31 17.4,23.57
  pour Route2 (isolate 0.254): 0,0 0,30.28 20.65,30.28 20.65,0
  pour Top (isolate 0.254, no thermals): 0.18,30.28 20.65,30.28 20.65,0 0,0 0,29.69
  pour Bottom (isolate 0.254, no thermals): 0,0 20.65,0 20.65,30.28 0,30.28 -0.03,24.56 0,24.56
LDOEN/D5  (via drill 0.25)
  Top 0.203: U6.P$37 8.77,24.87 v8.76,24.94
  Bottom 0.203: U8.P$3 12.91,26.48 R3.2 | 12.91,25.78 U8.P$3 | U8.P$3 12.84,25.73 10.24,25.76 9.3,24.94 v8.76,24.94
N$1
  Bottom 0.305: U2.P$4 L9.2
N$2
  Top 0.203: U6.P$45 9.76,17.47 10.01,17.22 10.01,15.24 9.8,15.04 8.8,15.04 U6.P$48
N$3
  Top 0.203: R9.2 U$4.P$2
N$4
  Top 0.203: U12.P$2 R20.2 | 13.06,4.19 R20.2 | R20.2 13.16,4.11 R21.2
N$5
  Bottom 0.254: L3.2 2.47,10.7
  Bottom 0.305: C10.2 RBIAS.2 2.47,10.7
N$6
  Top 0.254: U10.P$5 12.65,6.56 C14.2
N$7
  Bottom 0.203: U4.P$2 4.88,20.01 5.13,19.76 5.13,16.92 4.9,16.69 YELLOW.P$2
N$8
  Top 0.203: R14.1 7.05,22.02 U$5.P$2
N$10
  Top 0.203: U12.P$6 10.34,3.84 | U12.P$5 10.69,4.19 R22.1
  Top 0.254: 10.34,3.84 R22.1
N$11
  cutout Top: 16.87,9.32 20.14,9.32 20.14,6.02 16.87,6.02 16.87,9.3
N$12
  Top 0.203: U7.P$2 4.95,26.47 R13.2 R5.2
N$13
  Top 0.203: U7.P$5 2.95,26.47 R17.1 2.62,26.12 U7.P$6
N$14
  cutout Top: 0.43,10.87 6.25,10.87 6.25,4.45 0.43,4.45
N$15
  Bottom 0.203: R7.1 RED.P$1
N$16
  Top 0.305: 16.51,31.63 U$2.P$1
  Top 0.33: C95.1 16.51,31.63
N$17
  Bottom 0.203: R8.1 YELLOW.P$1
N$18
  Top 0.33: U13.P$3 16.34,29.33 C95.2
N$19
  Top 0.305: 15.52,28.07 U13.P$1
  Top 0.33: C103.1 15.63,27.42 15.52,27.53 15.52,28.07
N$20
  cutout Top: 17.83,29.69 20.45,29.69 20.45,27.1 17.83,27.1
N$22
  Top 0.203: R4.2 13.51,29.39 U13.P$4
N$23
  cutout Bottom: 0.36,8.56 2.92,8.56 2.92,5.97 0.36,5.97 0.36,8.53
N$27
  Bottom 0.203: U4.P$5 0.79,20.01 R18.2
N$43
  Bottom 0.305: U2.P$2 16.21,13.79 L4.2
N$44
  Bottom 0.305: U2.P$3 16.2,12.69 L5.2
PHO  (via drill 0.25)
  Top 0.203: U6.P$46 9.46,16.67 v9.55,16.71
  Bottom 0.203: U5.P$1 R1.1 12.93,20.73 11.99,20.73 11.43,20.17 11.43,17.32 10.82,16.71 v9.55,16.71
PPS/D4  (via drill 0.25)
  Top 0.203: U6.P$38 9.46,23.07 v9.55,23.19 | 8.75,23.09 U6.P$38 | U$5.P$1 8.53,22.98 U6.P$38
  Route2 0.203: v9.55,23.19 9.42,23.19 8.99,23.65 8.99,24.41 9.4,24.89 12.32,24.89 12.5,24.71 12.5,24.28 12.78,24 15.8,24 16.15,23.65 16.15,12.67 17.2,11.58 v17.88,11.58
  Bottom 0.203: L9.1 17.39,11.59 v17.88,11.58
PWRIN
  Bottom 0.305: U3.P$8 3.68,26.28 D1.P$1 | U3.P$7 3.73,25.78 3.65,25.83
  Bottom 0.406: D1.P$1 3.65,25.83 D2.P$1 3.65,24.67 C19.2
RF2
  Top 0.305: 16.52,28.4 C103.2
  Top 0.33: CONN3.P$3 16.52,28.4
RFIN
  Top 0.33: U6.P$26 17.57,26.43 C100.2
RFOUT
  Top 0.305: 16.32,26.54 C100.1
  Top 0.33: U13.P$5 14.2,28.73 14.33,28.6 14.33,28.19 14.96,27.56 14.96,26.95 15.37,26.54 16.32,26.54
RXD  (via drill 0.25)
  Top 0.203: U6.P$19 v18.41,19.87
  Route2 0.203: v18.41,19.87 17.1,19.87 16.59,19.35 16.59,13.38 L5.1 v17.88,12.7
  Bottom 0.203: v17.88,12.7 L5.1
SCL  (via drill 0.25)
  Top 0.203: U1.P$5 v11.25,7.67 | U10.P$1 12.13,8.46 12.13,8.8 v12.12,8.99 | R2.1 v9.5,10.79 | v17.98,9.55 17.98,9.04 U11.P$3 | U6.P$35 10.37,24.42 v10.39,24.36 | 5.32,10.96 5.49,11.14 5.49,11.78 4.88,12.45 v3.84,12.45
  Top 0.254: U9.P$1 5.32,10.96
  Route2 0.203: v9.5,10.79 9.5,11.1 9.7,11.28 10.9,11.28 11.3,11.68 11.3,23.44 v10.39,24.36
  Route15 0.203: v17.98,9.55 17.93,9.4 17.93,9.22 17.45,8.74 12.37,8.74 v12.12,8.99 11.3,8.99 | 11.3,8.99 10.16,8.99 9.5,9.65 v9.5,10.79 9.5,11.2 8.23,12.45 v3.84,12.45 | v11.25,7.67 11.25,8.94 11.3,8.99
SDA  (via drill 0.25)
  Top 0.203: U6.P$36 v9.57,24.36 v9.58,24.36 | U11.P$4 17.49,5.76 v17.5,5.66 | v11.56,6.91 12.1,6.91 U10.P$4 | R12.1 8.48,10.85 v8.53,10.82 | U9.P$7 4.18,4.15 v4.17,4.14 | U1.P$2 9.07,7.67 9.3,7.47 9.3,6.91 v9.55,6.63
  Route2 0.203: 11.53,6.27 11.58,6.2 12.34,5.44 17.27,5.44 v17.5,5.66 | v11.56,6.91 11.53,6.65 11.53,6.27 | 11.53,6.27 11.43,6.17 9.58,6.17 | 9.58,6.17 8.61,6.17 7.95,6.83 7.95,10.19 v8.53,10.82 9.4,11.68 10.69,11.68 10.9,11.86 10.9,23.04 v9.58,24.36 | v9.55,6.63 9.55,6.2 9.58,6.17
  Route15 0.203: v4.17,4.14 4.24,4.17 4.24,4.67 4.93,5.36 9.2,5.36 9.55,5.71 v9.55,6.63
SI  (via drill 0.25)
  Top 0.203: 19.15,15.85 U6.P$14 18.47,15.87 v18.41,15.9
  Bottom 0.203: U5.P$5 16.76,16.76 17.63,16.76 17.91,16.48 17.91,16.03 18.03,15.9 v18.41,15.9
SO  (via drill 0.25)
  Top 0.203: v18.41,16.69 19.15,16.69 U6.P$15
  Bottom 0.203: v18.41,16.69 18.82,16.69 18.9,16.76 18.9,17.72 18.66,17.93 15.85,17.93 15.19,18.59 15.19,20.69 U5.P$2
TRACE
  Top 0.254: 16.37,38.81 16.4,38.81 U$2.P$2
  Top 0.508: 16.37,38.81 4.34,38.81 4.34,37.79 14.43,37.79 14.43,36.78 4.34,36.78 4.34,35.76 11.61,35.76
TXD  (via drill 0.25)
  Top 0.203: U6.P$18 18.5,19.07 v18.41,19.15
  Route2 0.203: v18.41,19.15 17.37,19.15 16.99,18.77 16.99,14.91 v17.27,14.63
  Bottom 0.203: v17.27,14.63 17.27,13.83 L4.1
VBAT  (via drill 0.25)
  Top 0.203: U7.P$4 2.98,26.82 R17.2 2.42,27.08 1.56,27.08 JP9.1
  Route2 0.406: v5.18,22.4 4.01,22.4 3.61,22.81 3.61,25.54 JP9.1
  Bottom 0.406: U4.P$1 4.5,21.11 C24.1 v5.18,22.4 | D1.P$2 2.78,26.36 JP9.1
VBUS  (via drill 0.25)
  Top 0.203: v18.41,20.52 18.96,20.52 U6.P$20
  Route15 0.203: v18.41,20.52 15.75,20.52 15.39,20.14 15.39,18.64 14.86,18.08 6.66,18.08 5.94,18.87 v5.94,20.78 | 2.9,21.34 2.9,16.31 v2.44,15.85
  Route15 0.406: v2.9,24.46 2.9,22.35 | 2.9,22.35 2.9,21.34 3.45,20.78 v5.94,20.78 | v2.44,22.35 2.9,22.35
  Bottom 0.203: R7.2 R8.2 1.73,16.64 v2.44,15.85
  Bottom 0.406: v2.9,24.46 2.9,25.11 D2.P$2 | U4.P$6 1.58,21.14 C25.1 v2.44,22.35 | U$16.P$1 10.29,3.33 10.85,3.89 10.85,6.78 9.93,7.7 8.59,7.7 7.49,8.79 7.49,11.58 8.33,12.42 8.33,20.37 7.93,20.78 v5.94,20.78
VCC_RF
  Bottom 0.254: 4.75,10.72 3.63,10.72
  Bottom 0.305: U2.P$14 5.03,10.49 4.75,10.72 | 3.63,10.72 RBIAS.1

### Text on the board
tPlace: IoT Turtle / Tracker | 3V3 | D8 | D9 | + | BT | RST | - | A3 | 3V3 | GND | 3V3 | BTN | DP | 5V | DM | GND | -
bPlace: + | - | Pesky / Products | v.01b

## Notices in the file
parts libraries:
SparkFun-Connectors: Licensing: Creative Commons ShareAlike 4.0 International - https://creativecommons.org/licenses/by-sa/4.0
